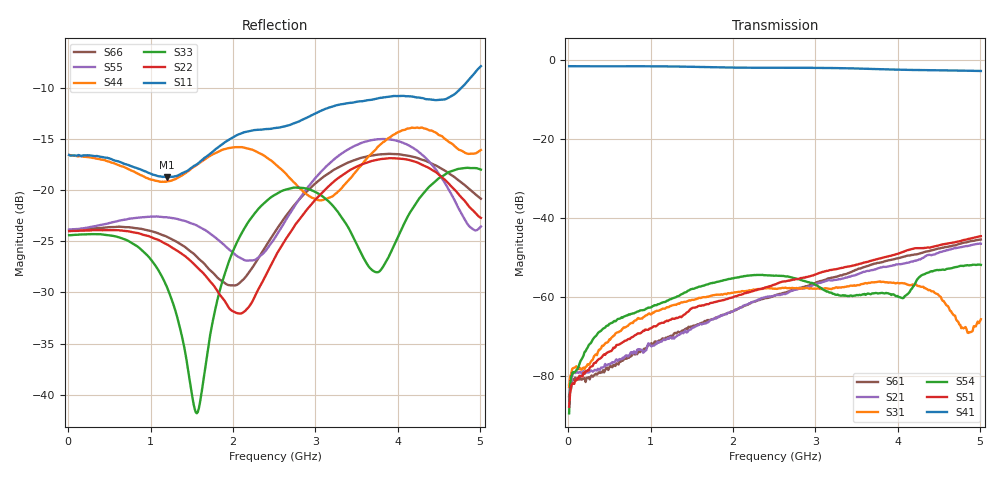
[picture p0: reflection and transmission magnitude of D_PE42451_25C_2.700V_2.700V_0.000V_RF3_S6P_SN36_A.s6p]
! Device ID: PE42451
! Serial: 36
! Insertion: A
! Temp: 25C
! VDD: 2.700
! Control_Hi: 100.000
! Control_Lo: 0.000
! Logic State: RF3
! Port 1: RFC
! Port 2: RF1
! Port 3: RF2
! Port 4: RF3
! Port 5: RF4
! Port 6: RF5
! V1 = 2.70
! V2 = 2.70
! V3 = 0.00
! V4 = 0.00
! IDD: 1.082870e-05
#  Hz  S  RI  R  50
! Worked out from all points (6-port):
!   401 points, 10 MHz to 5.01 GHz, reference 50 ohm
!   strongest paths, dB at 10 MHz, 1.26 GHz, 2.51 GHz, 3.76 GHz, 5.01 GHz:
!     S41: -1.5, -1.6, -1.9, -2.3, -2.7
!     S51: -87.8, -65.5, -56.8, -50.4, -44.6
!     S54: -89.5, -60.4, -54.6, -59.1, -51.9
!     S31: -82.8, -62.2, -57.9, -56.1, -65.7
!     S21: -82.3, -70.6, -59.6, -52.8, -46.5
!     S61: -85.2, -69.9, -59.6, -51.4, -45.4
!   lowest |S11| = -18.7 dB at 1.198 GHz (marker M1), VSWR 1.26, Z = 56.6 - j10.5 ohm
!   |S11| at or under -10 dB: start of sweep to 4.775 GHz
